|   stm32f427_437_429_439_ufbga169 IBIS Model
[IBIS ver]   4.2
[File name]  stm32f427_437_429_439_ufbga169.ibs
[File Rev]   1.3
[Date]   05-30-2014
[Source] Data Created at STMicroelectronics
[Notes]   File originated from ELDO simulations.
[Disclaimer]  This information is for modeling purpose only and is
   not guaranted. The information is subject to change without
   notice.
[Copyright] Copyright 2014 STMicroelectronics Inc.
[Component] stm32f427_437_429_439_ufbga169
[Manufacturer] STMicroelectronics
[Package]
| variable   typ   min   max
R_pkg   0.0   NA   NA
L_pkg   0.0H   NA   NA
C_pkg   0.0F   NA   NA
[Pin]   signal_name   model_name   R_pin   L_pin   C_pin
B2   PE2   io8p_arsudq_ft
C1   PE3   io8p_arsudq_ft
C2   PE4   io8p_arsudq_ft
D1   PE5   io8p_arsudq_ft
D2   PE6   io8p_arsudq_ft
E5   VBAT   POWER
|NC   PI8   io8p_arsudq_ft_v33
E4   PC13   io8p_arwsudq_ft_v33
E1   PC14   io8p_arwsudq_ft
F1   PC15   io8p_arsudq_ft
E2   PI9   io8p_arsudq_ft
E3   PI10   io8p_arsudq_ft
|NC   PI11   io8p_arsudq_ft
F6   VSS   GND
F4   VDD   POWER
F2   PF0   io8p_arsudq_i2cin_ft
F3   PF1   io8p_arsudq_i2cin_ft
G5   PF2   io8p_arsudq_ft
G4   PF3   io8p_arwsudq_ft
G3   PF4   io8p_arwsudq_ft
H3   PF5   io8p_arwsudq_ft
G7   VSS   GND
G8   VDD   POWER
|NC   PF6   io8p_arwsudq_ft
|NC   PF7   io8p_arwsudq_ft
|NC   PF8   io8p_arwsudq_ft
|NC   PF9   io8p_arwsudq_ft
H1   PF10   io8p_arwsudq_ft
G2   PH0   io8p_arsudq_ft
G1   PH1   io8p_arsudq_ft
H2   NRST   ioreset_ft_v33
G6   PC0   io8p_ar3wsudq_ft
H5   PC1   io8p_ar3wsudq_ft
H6   PC2   io8p_ar3wsudq_ft
H7   PC3   io8p_ar3wsudq_ft
J1   VSSA  GND
J2   VREFM   POWER
J3   VREFP   POWER
J4   VDDA   POWER
J5   PA0   io8p_ar3wsudq_ft_v33
K1   PA1   io8p_ar3wsudq_ft
K2   PA2   io8p_ar3wsudq_ft
L2   PH2   io8p_arsudq_ft
L1   PH3   io8p_arsudq_ft
M2   PH4   io8p_arsudq_i2cin_ft
L3   PH5   io8p_arsudq_i2cin_ft
K3   PA3   io8p_ar3wsudq_ft
M1   BYPASS_REG io8p_arsudq_ft_v33
J11   VDD   POWER
N2   PA4   io8p_ar3wsudq_ft
M3   PA5   io8p_ar3wsudq_ft
N3   PA6   io8p_ar3wsudq_ft
K4   PA7   io8p_ar3wsudq_ft
L4   PC4   io8p_ar3wsudq_ft
M4   PC5   io8p_ar3wsudq_ft
N4   PB0   io8p_ar3wsudq_ft
K5   PB1   io8p_ar3wsudq_ft
L5   PB2   io8p_ar3wsudq_ft
M5   PF11   io8p_arsudq_ft
N5   PF12   io8p_arsudq_ft
G9   VSS   GND
D10   VDD   POWER
M6   PF13   io8p_arsudq_ft
K7   PF14   io8p_arsudq_ft
L7   PF15   io8p_arsudq_ft
N6   PG0   io8p_arsudq_ft
M7   PG1   io8p_arsudq_ft
N7   PE7   io8p_arsudq_ft
J8   PE8   io8p_arsudq_ft
K8   PE9   io8p_arsudq_ft
J6   VSS   GND
G10   VDD   POWER
L8   PE10   io8p_arsudq_ft
M8   PE11   io8p_arsudq_ft
N8   PE12   io8p_arsudq_ft
H9   PE13   io8p_arsudq_ft
J9   PE14   io8p_arsudq_ft
K9   PE15   io8p_ar3wsudq_ft
L9   PB10   io8p_arsudq_i2cin_ft
M9   PB11   io8p_arsudq_i2cin_ft
N9   VCAP1   POWER
F8   VDD   POWER
N10   PH6   io8p_arsudq_ft
M10   PH7   io8p_arsudq_i2cin_ft
L10   PH8   io8p_arsudq_i2cin_ft
K10   PH9   io8p_arsudq_ft
N11   PH10   io8p_arsudq_ft
M11   PH11   io8p_arsudq_ft
L11   PH12   io8p_arsudq_ft
E7   VSS   GND
H8   VDD   POWER
N12   PB12   io8usb_id_otg_ft
M12   PB13   io8usb_vbus_otg_ft
M13   PB14   io8usb_lsfs_otg_ft
L13   PB15   io8usb_lsfs_otg_ft
L12   PD8   io8p_arsudq_ft
K13   PD9   io8p_arsudq_ft
K11   PD10   io8p_arsudq_ft
H10   PD11   io8p_arsudq_ft
J13   PD12   io8p_arsudq_ft
K12   PD13   io8p_arsudq_ft
F7   VDD   POWER
H11   PD14   io8p_arsudq_ft
J12   PD15   io8p_arsudq_ft
H13   PG2   io8p_arsudq_ft
|NC   PG3   io8p_arsudq_ft
H12   PG4   io8p_arsudq_ft
G13   PG5   io8p_arsudq_ft
G11   PG6   io8p_arsudq_ft
G12   PG7   io8p_arsudq_ft
F13   PG8   io8p_arsudq_ft
J7   VSS   GND
E6   VDD   POWER
F9   PC6   io8p_arsudq_ft
F10   PC7   io8p_arsudq_ft
F11   PC8   io8p_arsudq_ft
F12   PC9   io8p_arsudq_i2cin_ft
E13   PA8   io8p_arsudq_i2cin_ft
E8   PA9   io8usb_vbus_otg_ft
E9   PA10   io8usb_id_otg_ft
E10   PA11   io8usb_lsfs_otg_ft
E11   PA12   io8usb_lsfs_otg_ft
E12   PA13   io8p_arsudq_ft
D12   VCAP2   POWER
J10   VSS   GND
H4   VDD   POWER
D13   PH13   io8p_arsudq_ft
C13   PH14   io8p_arsudq_ft
C12   PH15   io8p_arsudq_ft
B13   PI0   io8p_arsudq_ft
C11   PI1   io8p_arsudq_ft
B12   PI2   io8p_arsudq_ft
A12   PI3   io8p_arsudq_ft
D11   VSS   GND
D3   VDD   POWER
A11   PA14   io8p_arsudq_ft
B11   PA15   io8p_arsudq_ft
C10   PC10   io8p_arsudq_ft
B10   PC11   io8p_arsudq_ft
A10   PC12   io8p_arsudq_ft
D9   PD0   io8p_arsudq_ft
C9   PD1   io8p_arsudq_ft
B9   PD2   io8p_arsudq_ft
A9   PD3   io8p_arsudq_ft
D8   PD4   io8p_arsudq_ft
C8   PD5   io8p_arsudq_ft
D6   VDD   POWER
B8   PD6   io8p_arsudq_ft
A8   PD7   io8p_arsudq_ft
|NC   PG9   io8p_arsudq_ft
C7   PG10   io8p_arsudq_ft
B7   PG11   io8p_arsudq_ft
A7   PG12   io8p_arsudq_ft
|NC   PG13   io8p_arsudq_ft
|NC   PG14   io8p_arsudq_ft
D7   VSS   GND
L6   VDD   POWER
C6   PG15   io8p_arsudq_ft
B6   PB3   io8p_arsudq_ft
A6   PB4   io8p_arsudq_ft
D5   PB5   io8p_ar3wsudq_ft
C5   PB6   io8p_arsudq_i2cin_ft
B5   PB7   io8p_arsudq_i2cin_ft
A5   BOOT0   vpp_test_hv
D4   PB8   io8p_arsudq_i2cin_ft
C4   PB9   io8p_arsudq_i2cin_ft
B4   PE0   io8p_arsudq_ft
A4   PE1   io8p_arsudq_ft
F5   VSS   GND
C3   PDR_ON   io8p_arsudq_ft_v33
K6   VDD   POWER
B3   PI4   io8p_arsudq_ft
A3   PI5   io8p_arsudq_ft
A2   PI6   io8p_arsudq_ft
B1   PI7   io8p_arsudq_ft
[Diff Pin]   inv_pin   vdiff   tdelay_typ  tdelay_min  tdelay_max
M13   L13   200mV   NA   NA   NA
E11   E10   200mV   NA   NA   NA
[Model Selector] io8p_ar3wsudq_ft
io8p00_ar3wsudq_ft_pd_lv  "SPEED00 1P8V, PD=40kOhm"
io8p00_ar3wsudq_ft_pu_lv  "SPEED00 1P8V, PU=40kOhm"
io8p00_ar3wsudq_ft_lv   "SPEED00 1P8V"
io8p01_ar3wsudq_ft_pd_lv  "SPEED01 1P8V, PD=40kOhm"
io8p01_ar3wsudq_ft_pu_lv  "SPEED01 1P8V, PU=40kOhm"
io8p01_ar3wsudq_ft_lv  "SPEED01 1P8V"
io8p10_ar3wsudq_ft_pd_lv  "SPEED10 1P8V, PD=40kOhm"
io8p10_ar3wsudq_ft_pu_lv  "SPEED10 1P8V, PU=40kOhm"
io8p10_ar3wsudq_ft_lv  "SPEED10 1P8V"
io8p11_ar3wsudq_ft_pd_lv  "SPEED11 1P8V, PD=40kOhm"
io8p11_ar3wsudq_ft_pu_lv  "SPEED11 1P8V, PU=40kOhm"
io8p11_ar3wsudq_ft_lv  "SPEED11 1P8V"
io8p00_ar3wsudq_ft_pd  "SPEED00, PD=40kOhm"
io8p00_ar3wsudq_ft_pu  "SPEED00, PU=40kOhm"
io8p00_ar3wsudq_ft  "SPEED00"
io8p01_ar3wsudq_ft_pd  "SPEED01, PD=40kOhm"
io8p01_ar3wsudq_ft_pu  "SPEED01, PU=40kOhm"
io8p01_ar3wsudq_ft  "SPEED01"
io8p10_ar3wsudq_ft_pd  "SPEED10, PD=40kOhm"
io8p10_ar3wsudq_ft_pu  "SPEED10, PU=40kOhm"
io8p10_ar3wsudq_ft  "SPEED10"
io8p11_ar3wsudq_ft_pd  "SPEED11, PD=40kOhm"
io8p11_ar3wsudq_ft_pu  "SPEED11, PU=40kOhm"
io8p11_ar3wsudq_ft  "SPEED11"
[Model Selector] io8p_ar3wsudq_ft_v33
io8p00_ar3wsudq_ft_v33_pd_lv  "SPEED00 1P8V, PD=40kOhm"
io8p00_ar3wsudq_ft_v33_pu_lv  "SPEED00 1P8V, PU=40kOhm"
io8p00_ar3wsudq_ft_v33_lv  "SPEED00 1P8V"
io8p01_ar3wsudq_ft_v33_pd_lv  "SPEED01 1P8V, PD=40kOhm"
io8p01_ar3wsudq_ft_v33_pu_lv  "SPEED01 1P8V, PU=40kOhm"
io8p01_ar3wsudq_ft_v33_lv  "SPEED01 1P8V"
io8p10_ar3wsudq_ft_v33_pd_lv  "SPEED10 1P8V, PD=40kOhm"
io8p10_ar3wsudq_ft_v33_pu_lv  "SPEED10 1P8V, PU=40kOhm"
io8p10_ar3wsudq_ft_v33_lv  "SPEED10 1P8V"
io8p11_ar3wsudq_ft_v33_pd_lv  "SPEED11 1P8V, PD=40kOhm"
io8p11_ar3wsudq_ft_v33_pu_lv  "SPEED11 1P8V, PU=40kOhm"
io8p11_ar3wsudq_ft_v33_lv  "SPEED11 1P8V"
io8p00_ar3wsudq_ft_v33_pd  "SPEED00, PD=40kOhm"
io8p00_ar3wsudq_ft_v33_pu  "SPEED00, PU=40kOhm"
io8p00_ar3wsudq_ft_v33  "SPEED00"
io8p01_ar3wsudq_ft_v33_pd  "SPEED01, PD=40kOhm"
io8p01_ar3wsudq_ft_v33_pu  "SPEED01, PU=40kOhm"
io8p01_ar3wsudq_ft_v33  "SPEED01"
io8p10_ar3wsudq_ft_v33_pd  "SPEED10, PD=40kOhm"
io8p10_ar3wsudq_ft_v33_pu  "SPEED10, PU=40kOhm"
io8p10_ar3wsudq_ft_v33  "SPEED10"
io8p11_ar3wsudq_ft_v33_pd  "SPEED11, PD=40kOhm"
io8p11_ar3wsudq_ft_v33_pu  "SPEED11, PU=40kOhm"
io8p11_ar3wsudq_ft_v33  "SPEED11"
[Model Selector] io8p_arsudq_ft
io8p00_arsudq_ft_pd_lv  "SPEED00 1P8V, PD=40kOhm"
io8p00_arsudq_ft_pu_lv  "SPEED00 1P8V, PU=40kOhm"
io8p00_arsudq_ft_lv  "SPEED00 1P8V"
io8p01_arsudq_ft_pd_lv  "SPEED01 1P8V, PD=40kOhm"
io8p01_arsudq_ft_pu_lv  "SPEED01 1P8V, PU=40kOhm"
io8p01_arsudq_ft_lv  "SPEED01 1P8V"
io8p10_arsudq_ft_pd_lv  "SPEED10 1P8V, PD=40kOhm"
io8p10_arsudq_ft_pu_lv  "SPEED10 1P8V, PU=40kOhm"
io8p10_arsudq_ft_lv  "SPEED10 1P8V"
io8p11_arsudq_ft_pd_lv  "SPEED11 1P8V, PD=40kOhm"
io8p11_arsudq_ft_pu_lv  "SPEED11 1P8V, PU=40kOhm"
io8p11_arsudq_ft_lv  "SPEED11 1P8V"
io8p00_arsudq_ft_pd  "SPEED00, PD=40kOhm"
io8p00_arsudq_ft_pu  "SPEED00, PU=40kOhm"
io8p00_arsudq_ft  "SPEED00"
io8p01_arsudq_ft_pd  "SPEED01, PD=40kOhm"
io8p01_arsudq_ft_pu  "SPEED01, PU=40kOhm"
io8p01_arsudq_ft  "SPEED01"
io8p10_arsudq_ft_pd  "SPEED10, PD=40kOhm"
io8p10_arsudq_ft_pu  "SPEED10, PU=40kOhm"
io8p10_arsudq_ft  "SPEED10"
io8p11_arsudq_ft_pd  "SPEED11, PD=40kOhm"
io8p11_arsudq_ft_pu  "SPEED11, PU=40kOhm"
io8p11_arsudq_ft  "SPEED11"
[Model Selector] io8p_arsudq_ft_v33
io8p00_arsudq_ft_v33_pd_lv  "SPEED00 1P8V, PD=40kOhm"
io8p00_arsudq_ft_v33_pu_lv  "SPEED00 1P8V, PU=40kOhm"
io8p00_arsudq_ft_v33_lv  "SPEED00 1P8V"
io8p01_arsudq_ft_v33_pd_lv  "SPEED01 1P8V, PD=40kOhm"
io8p01_arsudq_ft_v33_pu_lv  "SPEED01 1P8V, PU=40kOhm"
io8p01_arsudq_ft_v33_lv  "SPEED01 1P8V"
io8p10_arsudq_ft_v33_pd_lv  "SPEED10 1P8V, PD=40kOhm"
io8p10_arsudq_ft_v33_pu_lv  "SPEED10 1P8V, PU=40kOhm"
io8p10_arsudq_ft_v33_lv  "SPEED10 1P8V"
io8p11_arsudq_ft_v33_pd_lv  "SPEED11 1P8V, PD=40kOhm"
io8p11_arsudq_ft_v33_pu_lv  "SPEED11 1P8V, PU=40kOhm"
io8p11_arsudq_ft_v33_lv  "SPEED11 1P8V"
io8p00_arsudq_ft_v33_pd  "SPEED00, PD=40kOhm"
io8p00_arsudq_ft_v33_pu  "SPEED00, PU=40kOhm"
io8p00_arsudq_ft_v33  "SPEED00"
io8p01_arsudq_ft_v33_pd  "SPEED01, PD=40kOhm"
io8p01_arsudq_ft_v33_pu  "SPEED01, PU=40kOhm"
io8p01_arsudq_ft_v33  "SPEED01"
io8p10_arsudq_ft_v33_pd  "SPEED10, PD=40kOhm"
io8p10_arsudq_ft_v33_pu  "SPEED10, PU=40kOhm"
io8p10_arsudq_ft_v33  "SPEED10"
io8p11_arsudq_ft_v33_pd  "SPEED11, PD=40kOhm"
io8p11_arsudq_ft_v33_pu  "SPEED11, PU=40kOhm"
io8p11_arsudq_ft_v33  "SPEED11"
[Model Selector] io8p_arsudq_i2cin_ft
io8p00_arsudq_i2cin_ft_pd_lv  "SPEED00 1P8V, PD=40kOhm"
io8p00_arsudq_i2cin_ft_pu_lv  "SPEED00 1P8V, PU=40kOhm"
io8p00_arsudq_i2cin_ft_lv  "SPEED00 1P8V"
io8p01_arsudq_i2cin_ft_pd_lv  "SPEED01 1P8V, PD=40kOhm"
io8p01_arsudq_i2cin_ft_pu_lv  "SPEED01 1P8V, PU=40kOhm"
io8p01_arsudq_i2cin_ft_lv  "SPEED01 1P8V"
io8p10_arsudq_i2cin_ft_pd_lv  "SPEED10 1P8V, PD=40kOhm"
io8p10_arsudq_i2cin_ft_pu_lv  "SPEED10 1P8V, PU=40kOhm"
io8p10_arsudq_i2cin_ft_lv  "SPEED10 1P8V"
io8p11_arsudq_i2cin_ft_pd_lv  "SPEED11 1P8V, PD=40kOhm"
io8p11_arsudq_i2cin_ft_pu_lv  "SPEED11 1P8V, PU=40kOhm"
io8p11_arsudq_i2cin_ft_lv  "SPEED11 1P8V"
io8p00_arsudq_i2cin_ft_pd  "SPEED00, PD=40kOhm"
io8p00_arsudq_i2cin_ft_pu  "SPEED00, PU=40kOhm"
io8p00_arsudq_i2cin_ft  "SPEED00"
io8p01_arsudq_i2cin_ft_pd  "SPEED01, PD=40kOhm"
io8p01_arsudq_i2cin_ft_pu  "SPEED01, PU=40kOhm"
io8p01_arsudq_i2cin_ft  "SPEED01"
io8p10_arsudq_i2cin_ft_pd  "SPEED10, PD=40kOhm"
io8p10_arsudq_i2cin_ft_pu  "SPEED10, PU=40kOhm"
io8p10_arsudq_i2cin_ft  "SPEED10"
io8p11_arsudq_i2cin_ft_pd  "SPEED11, PD=40kOhm"
io8p11_arsudq_i2cin_ft_pu  "SPEED11, PU=40kOhm"
io8p11_arsudq_i2cin_ft  "SPEED11"
[Model Selector] io8p_arwsudq_ft
io8p00_arwsudq_ft_pd_lv  "SPEED00 1P8V, PD=40kOhm"
io8p00_arwsudq_ft_pu_lv  "SPEED00 1P8V, PU=40kOhm"
io8p00_arwsudq_ft_lv  "SPEED00 1P8V"
io8p01_arwsudq_ft_pd_lv  "SPEED01 1P8V, PD=40kOhm"
io8p01_arwsudq_ft_pu_lv  "SPEED01 1P8V, PU=40kOhm"
io8p01_arwsudq_ft_lv  "SPEED01 1P8V"
io8p10_arwsudq_ft_pd_lv  "SPEED10 1P8V, PD=40kOhm"
io8p10_arwsudq_ft_pu_lv  "SPEED10 1P8V, PU=40kOhm"
io8p10_arwsudq_ft_lv  "SPEED10 1P8V"
io8p11_arwsudq_ft_pd_lv  "SPEED11 1P8V, PD=40kOhm"
io8p11_arwsudq_ft_pu_lv  "SPEED11 1P8V, PU=40kOhm"
io8p11_arwsudq_ft_lv  "SPEED11 1P8V"
io8p00_arwsudq_ft_pd  "SPEED00, PD=40kOhm"
io8p00_arwsudq_ft_pu  "SPEED00, PU=40kOhm"
io8p00_arwsudq_ft  "SPEED00"
io8p01_arwsudq_ft_pd  "SPEED01, PD=40kOhm"
io8p01_arwsudq_ft_pu  "SPEED01, PU=40kOhm"
io8p01_arwsudq_ft  "SPEED01"
io8p10_arwsudq_ft_pd  "SPEED10, PD=40kOhm"
io8p10_arwsudq_ft_pu  "SPEED10, PU=40kOhm"
io8p10_arwsudq_ft  "SPEED10"
io8p11_arwsudq_ft_pd  "SPEED11, PD=40kOhm"
io8p11_arwsudq_ft_pu  "SPEED11, PU=40kOhm"
io8p11_arwsudq_ft  "SPEED11"
[Model Selector] io8p_arwsudq_ft_v33
io8p00_arwsudq_ft_v33_pd_lv  "SPEED00 1P8V, PD=40kOhm"
io8p00_arwsudq_ft_v33_pu_lv  "SPEED00 1P8V, PU=40kOhm"
io8p00_arwsudq_ft_v33_lv  "SPEED00 1P8V"
io8p01_arwsudq_ft_v33_pd_lv  "SPEED01 1P8V, PD=40kOhm"
io8p01_arwsudq_ft_v33_pu_lv  "SPEED01 1P8V, PU=40kOhm"
io8p01_arwsudq_ft_v33_lv  "SPEED01 1P8V"
io8p10_arwsudq_ft_v33_pd_lv  "SPEED10 1P8V, PD=40kOhm"
io8p10_arwsudq_ft_v33_pu_lv  "SPEED10 1P8V, PU=40kOhm"
io8p10_arwsudq_ft_v33_lv  "SPEED10 1P8V"
io8p11_arwsudq_ft_v33_pd_lv  "SPEED11 1P8V, PD=40kOhm"
io8p11_arwsudq_ft_v33_pu_lv  "SPEED11 1P8V, PU=40kOhm"
io8p11_arwsudq_ft_v33_lv  "SPEED11 1P8V"
io8p00_arwsudq_ft_v33_pd  "SPEED00, PD=40kOhm"
io8p00_arwsudq_ft_v33_pu  "SPEED00, PU=40kOhm"
io8p00_arwsudq_ft_v33  "SPEED00"
io8p01_arwsudq_ft_v33_pd  "SPEED01, PD=40kOhm"
io8p01_arwsudq_ft_v33_pu  "SPEED01, PU=40kOhm"
io8p01_arwsudq_ft_v33  "SPEED01"
io8p10_arwsudq_ft_v33_pd  "SPEED10, PD=40kOhm"
io8p10_arwsudq_ft_v33_pu  "SPEED10, PU=40kOhm"
io8p10_arwsudq_ft_v33  "SPEED10"
io8p11_arwsudq_ft_v33_pd  "SPEED11, PD=40kOhm"
io8p11_arwsudq_ft_v33_pu  "SPEED11, PU=40kOhm"
io8p11_arwsudq_ft_v33  "SPEED11"
[Model Selector] io8usb_id_otg_ft
io8p00_id_otg_ft_pd_lv  "SPEED00 1P8V, PD=14kOhm"
io8p00_id_otg_ft_pu_lv  "SPEED00 1P8V, PU=14kOhm"
io8p00_id_otg_ft_lv  "SPEED00 1P8V"
io8p01_id_otg_ft_pd_lv  "SPEED01 1P8V, PD=14kOhm"
io8p01_id_otg_ft_pu_lv  "SPEED01 1P8V, PU=14kOhm"
io8p01_id_otg_ft_lv  "SPEED01 1P8V"
io8p10_id_otg_ft_pd_lv  "SPEED10 1P8V, PD=14kOhm"
io8p10_id_otg_ft_pu_lv  "SPEED10 1P8V, PU=14kOhm"
io8p10_id_otg_ft_lv  "SPEED10 1P8V"
io8p11_id_otg_ft_pd_lv  "SPEED11 1P8V, PD=14kOhm"
io8p11_id_otg_ft_pu_lv  "SPEED11 1P8V, PU=14kOhm"
io8p11_id_otg_ft_lv  "SPEED11 1P8V"
io8p00_id_otg_ft_pd  "SPEED00, PD=14kOhm"
io8p00_id_otg_ft_pu  "SPEED00, PU=14kOhm"
io8p00_id_otg_ft  "SPEED00"
io8p01_id_otg_ft_pd  "SPEED01, PD=14kOhm"
io8p01_id_otg_ft_pu  "SPEED01, PU=14kOhm"
io8p01_id_otg_ft  "SPEED01"
io8p10_id_otg_ft_pd  "SPEED10, PD=14kOhm"
io8p10_id_otg_ft_pu  "SPEED10, PU=14kOhm"
io8p10_id_otg_ft  "SPEED10"
io8p11_id_otg_ft_pd  "SPEED11, PD=14kOhm"
io8p11_id_otg_ft_pu  "SPEED11, PU=14kOhm"
io8p11_id_otg_ft  "SPEED11"
[Model Selector] io8usb_lsfs_otg_ft
io8usb_ls_otg_ft_dpdn_pd  "LS USB DP/DN IO + PD=20kOhm"
io8usb_ls_otg_ft_dpdn_pupu2  "LS USB DP/DN IO + PU/PU2=2.2kOhm"
io8usb_ls_otg_ft_dpdn_pu2  "LS USB DP/DN IO + PU2=1.2kOhm"
io8usb_ls_otg_ft_dpdn_pu  "LS USB DP/DN IO + PU=1.2kOhm"
io8usb_ls_otg_ft_dpdn  "LS USB DP/DN IO"
io8usb_fs_otg_ft_dpdn_pd  "HS USB DP/DN IO + PD=20kOhm"
io8usb_fs_otg_ft_dpdn_pupu2  "HS USB DP/DN IO + PU/PU2=2.2kOhm"
io8usb_fs_otg_ft_dpdn_pu2  "HS USB DP/DN IO + PU2=1.2kOhm"
io8usb_fs_otg_ft_dpdn_pu  "HS USB DP/DN IO + PU=1.2kOhm"
io8usb_fs_otg_ft_dpdn  "HS USB DP/DN IO"
io8p00_lsfs_otg_ft_pd_lv  "SPEED00 1P8V, PD=40kOhm"
io8p00_lsfs_otg_ft_pu_lv  "SPEED00 1P8V, PU=40kOhm"
io8p00_lsfs_otg_ft_lv  "SPEED00 1P8V"
io8p01_lsfs_otg_ft_pd_lv  "SPEED01 1P8V, PD=40kOhm"
io8p01_lsfs_otg_ft_pu_lv  "SPEED01 1P8V, PU=40kOhm"
io8p01_lsfs_otg_ft_lv  "SPEED01 1P8V"
io8p10_lsfs_otg_ft_pd_lv  "SPEED10 1P8V, PD=40kOhm"
io8p10_lsfs_otg_ft_pu_lv  "SPEED10 1P8V, PU=40kOhm"
io8p10_lsfs_otg_ft_lv  "SPEED10 1P8V"
io8p11_lsfs_otg_ft_pd_lv  "SPEED11 1P8V, PD=40kOhm"
io8p11_lsfs_otg_ft_pu_lv  "SPEED11 1P8V, PU=40kOhm"
io8p11_lsfs_otg_ft_lv  "SPEED11 1P8V"
io8p00_lsfs_otg_ft_pd  "SPEED00, PD=40kOhm"
io8p00_lsfs_otg_ft_pu  "SPEED00, PU=40kOhm"
io8p00_lsfs_otg_ft  "SPEED00"
io8p01_lsfs_otg_ft_pd  "SPEED01, PD=40kOhm"
io8p01_lsfs_otg_ft_pu  "SPEED01, PU=40kOhm"
io8p01_lsfs_otg_ft  "SPEED01"
io8p10_lsfs_otg_ft_pd  "SPEED10, PD=40kOhm"
io8p10_lsfs_otg_ft_pu  "SPEED10, PU=40kOhm"
io8p10_lsfs_otg_ft  "SPEED10"
io8p11_lsfs_otg_ft_pd  "SPEED11, PD=40kOhm"
io8p11_lsfs_otg_ft_pu  "SPEED11, PU=40kOhm"
io8p11_lsfs_otg_ft  "SPEED11"
[Model Selector] io8usb_vbus_otg_ft
io8psenb_vbus_otg_ft  "VBUS PULSE, SENSE VB"
io8psenab_vbus_otg_ft  "VBUS PULSE, SENSE VA and VB"
io8psena_vbus_otg_ft  "VBUS PULSE, SENSE VA"
io8psen_vbus_otg_ft  "VBUS PULSE"
io8p00_vbus_otg_ft_pd_lv  "SPEED00 1P8V, PD=40kOhm"
io8p00_vbus_otg_ft_pu_lv  "SPEED00 1P8V, PU=40kOhm"
io8p00_vbus_otg_ft_lv  "SPEED00 1P8V"
io8p01_vbus_otg_ft_pd_lv  "SPEED01 1P8V, PD=40kOhm"
io8p01_vbus_otg_ft_pu_lv  "SPEED01 1P8V, PU=40kOhm"
io8p01_vbus_otg_ft_lv  "SPEED01 1P8V"
io8p10_vbus_otg_ft_pd_lv  "SPEED10 1P8V, PD=40kOhm"
io8p10_vbus_otg_ft_pu_lv  "SPEED10 1P8V, PU=40kOhm"
io8p10_vbus_otg_ft_lv  "SPEED10 1P8V"
io8p11_vbus_otg_ft_pd_lv  "SPEED11 1P8V, PD=40kOhm"
io8p11_vbus_otg_ft_pu_lv  "SPEED11 1P8V, PU=40kOhm"
io8p11_vbus_otg_ft_lv  "SPEED11 1P8V"
io8p00_vbus_otg_ft_pd  "SPEED00, PD=40kOhm"
io8p00_vbus_otg_ft_pu  "SPEED00, PU=40kOhm"
io8p00_vbus_otg_ft  "SPEED00"
io8p01_vbus_otg_ft_pd  "SPEED01, PD=40kOhm"
io8p01_vbus_otg_ft_pu  "SPEED01, PU=40kOhm"
io8p01_vbus_otg_ft  "SPEED01"
io8p10_vbus_otg_ft_pd  "SPEED10, PD=40kOhm"
io8p10_vbus_otg_ft_pu  "SPEED10, PU=40kOhm"
io8p10_vbus_otg_ft  "SPEED10"
io8p11_vbus_otg_ft_pd  "SPEED11, PD=40kOhm"
io8p11_vbus_otg_ft_pu  "SPEED11, PU=40kOhm"
io8p11_vbus_otg_ft  "SPEED11"
[Model Selector] ioreset_ft_v33
ioreset_ft_v33_pu_lv  "ioreset 1P8V + PU=40kOhm"
ioreset_ft_v33_nopu_lv  "ioreset 1P8V"
ioreset_ft_v33_pu  "ioreset + PU=40kOhm"
ioreset_ft_v33_nopu  "ioreset"
[Model Selector] vpp_test_hv
vpp_test_hv_2p4  "Input Buffer 1P8V"
vpp_test_hv_3p3  "Input Buffer"
| Models and submodels in the file (260): io8p00_ar3wsudq_ft_pd_lv (I/O), io8p00_ar3wsudq_ft_pu_lv (I/O), io8p00_ar3wsudq_ft_lv (I/O), io8p01_ar3wsudq_ft_pd_lv (I/O), io8p01_ar3wsudq_ft_pu_lv (I/O), io8p01_ar3wsudq_ft_lv (I/O), io8p10_ar3wsudq_ft_pd_lv (I/O), io8p10_ar3wsudq_ft_pu_lv (I/O), io8p10_ar3wsudq_ft_lv (I/O), io8p11_ar3wsudq_ft_pd_lv (I/O), io8p11_ar3wsudq_ft_pu_lv (I/O), io8p11_ar3wsudq_ft_lv (I/O), io8p00_ar3wsudq_ft_pd (I/O), io8p00_ar3wsudq_ft_pu (I/O), io8p00_ar3wsudq_ft (I/O), io8p01_ar3wsudq_ft_pd (I/O), io8p01_ar3wsudq_ft_pu (I/O), io8p01_ar3wsudq_ft (I/O), io8p10_ar3wsudq_ft_pd (I/O), io8p10_ar3wsudq_ft_pu (I/O), io8p10_ar3wsudq_ft (I/O), io8p11_ar3wsudq_ft_pd (I/O), io8p11_ar3wsudq_ft_pu (I/O), io8p11_ar3wsudq_ft (I/O), io8p00_ar3wsudq_ft_v33_pd_lv (I/O), io8p00_ar3wsudq_ft_v33_pu_lv (I/O), io8p00_ar3wsudq_ft_v33_lv (I/O), io8p01_ar3wsudq_ft_v33_pd_lv (I/O), io8p01_ar3wsudq_ft_v33_pu_lv (I/O), io8p01_ar3wsudq_ft_v33_lv (I/O), io8p10_ar3wsudq_ft_v33_pd_lv (I/O), io8p10_ar3wsudq_ft_v33_pu_lv (I/O), io8p10_ar3wsudq_ft_v33_lv (I/O), io8p11_ar3wsudq_ft_v33_pd_lv (I/O), io8p11_ar3wsudq_ft_v33_pu_lv (I/O), io8p11_ar3wsudq_ft_v33_lv (I/O), io8p00_ar3wsudq_ft_v33_pd (I/O), io8p00_ar3wsudq_ft_v33_pu (I/O), io8p00_ar3wsudq_ft_v33 (I/O), io8p01_ar3wsudq_ft_v33_pd (I/O), io8p01_ar3wsudq_ft_v33_pu (I/O), io8p01_ar3wsudq_ft_v33 (I/O), io8p10_ar3wsudq_ft_v33_pd (I/O), io8p10_ar3wsudq_ft_v33_pu (I/O), io8p10_ar3wsudq_ft_v33 (I/O), io8p11_ar3wsudq_ft_v33_pd (I/O), io8p11_ar3wsudq_ft_v33_pu (I/O), io8p11_ar3wsudq_ft_v33 (I/O), io8p00_arsudq_ft_pd_lv (I/O), io8p00_arsudq_ft_pu_lv (I/O), io8p00_arsudq_ft_lv (I/O), io8p01_arsudq_ft_pd_lv (I/O), io8p01_arsudq_ft_pu_lv (I/O), io8p01_arsudq_ft_lv (I/O), io8p10_arsudq_ft_pd_lv (I/O), io8p10_arsudq_ft_pu_lv (I/O), io8p10_arsudq_ft_lv (I/O), io8p11_arsudq_ft_pd_lv (I/O), io8p11_arsudq_ft_pu_lv (I/O), io8p11_arsudq_ft_lv (I/O), io8p00_arsudq_ft_pd (I/O), io8p00_arsudq_ft_pu (I/O), io8p00_arsudq_ft (I/O), io8p01_arsudq_ft_pd (I/O), io8p01_arsudq_ft_pu (I/O), io8p01_arsudq_ft (I/O), io8p10_arsudq_ft_pd (I/O), io8p10_arsudq_ft_pu (I/O), io8p10_arsudq_ft (I/O), io8p11_arsudq_ft_pd (I/O), io8p11_arsudq_ft_pu (I/O), io8p11_arsudq_ft (I/O), io8p00_arsudq_ft_v33_pd_lv (I/O), io8p00_arsudq_ft_v33_pu_lv (I/O), io8p00_arsudq_ft_v33_lv (I/O), io8p01_arsudq_ft_v33_pd_lv (I/O), io8p01_arsudq_ft_v33_pu_lv (I/O), io8p01_arsudq_ft_v33_lv (I/O), io8p10_arsudq_ft_v33_pd_lv (I/O), io8p10_arsudq_ft_v33_pu_lv (I/O)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
